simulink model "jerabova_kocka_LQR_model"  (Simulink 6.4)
settings: Solver=ode45  StartTime=0.0  StopTime=250  RelTol=1e-3
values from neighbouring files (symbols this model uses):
  A = [0 1 0 0 0    [kockaLQG.m]    (also in kockaLQR.m; podklad.m = [dh1_h10 dh1_h20 0; testx.m = [ -0.195 0.195; 0.195 -0.205]; kulicka_na_tyci_LQG_podklad.m = [0 0;1 0])
  B = [0    [kockaLQG.m]    (also in kockaLQR.m; podklad.m = [dh1_q0; testx.m = [0.0047; 0]; kulicka_na_tyci_LQG_podklad.m = [7.14;0])
  C = [1 0 0 0 0]    [kockaLQG.m]    (also in kockaLQR.m; podklad.m = [0 0 1]; testx.m = [0 1]; kulicka_na_tyci_LQG_podklad.m = [0 1])
  K = tf(num,den)    [phinf2.m]
  Ng = lqr_kompenzace(A,B,C,D,K)    [kockaLQG.m]    (also in kockaLQR.m; lqr_kompenzace.m = Nu + K*Nx; testx.m; kulicka_na_tyci_LQG_podklad.m)

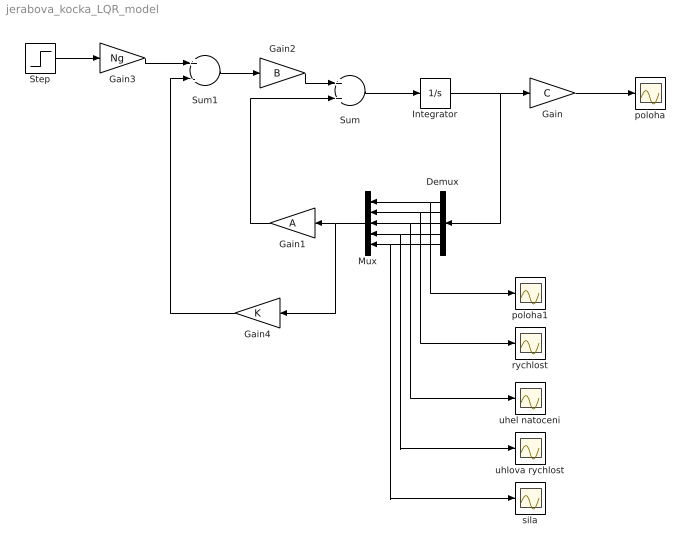
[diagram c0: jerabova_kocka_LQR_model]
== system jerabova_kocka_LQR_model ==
  Demux : Demux  Orientation=left  Outputs=5
  Gain : Gain  Gain=C  Multiplication=Matrix(K*u)
  Gain1 : Gain  Orientation=left  Gain=A  Multiplication=Matrix(K*u)
  Gain2 : Gain  Gain=B  Multiplication=Matrix(K*u)
  Gain3 : Gain  Gain=Ng
  Gain4 : Gain  Orientation=left  Gain=K  Multiplication=Matrix(K*u)
  Integrator : Integrator
  Mux : Mux  Orientation=left  Inputs=5
  Step : Step  Time=0  SampleTime=0
  Sum : Sum
  Sum1 : Sum  Inputs=+-
  poloha : Scope
  poloha1 : Scope
  rychlost : Scope
  sila : Scope
  uhel natoceni : Scope
  uhlova rychlost : Scope
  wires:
  Sum/1 -> Integrator/1
  Integrator/1 -> Gain/1, Demux/1
  Gain1/1 -> Sum/2
  Gain2/1 -> Sum/1
  Gain3/1 -> Sum1/1
  Step/1 -> Gain3/1
  Gain4/1 -> Sum1/2
  Sum1/1 -> Gain2/1
  Gain/1 -> poloha/1
  Mux/1 -> Gain1/1, Gain4/1
  Demux/1 -> Mux/1, poloha1/1
  Demux/2 -> Mux/2, rychlost/1
  Demux/3 -> Mux/3, uhel natoceni/1
  Demux/4 -> Mux/4, uhlova rychlost/1
  Demux/5 -> Mux/5, sila/1
